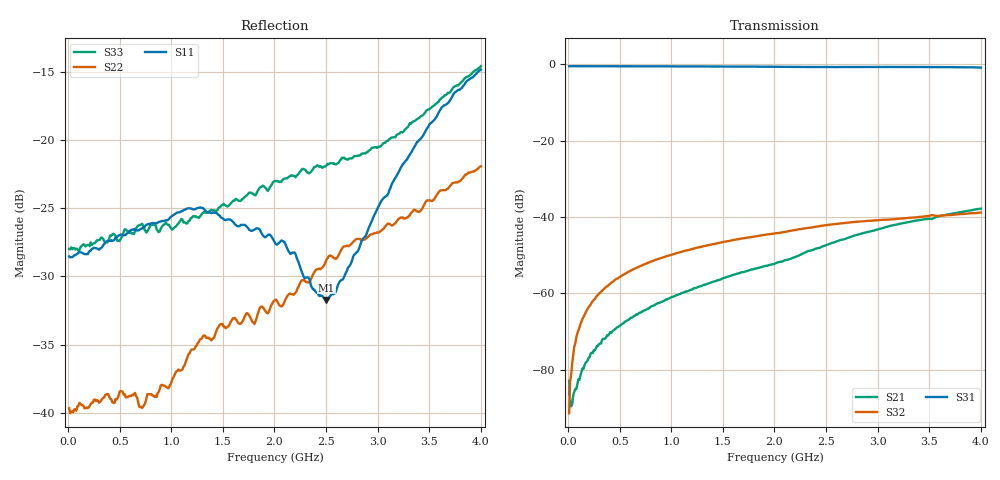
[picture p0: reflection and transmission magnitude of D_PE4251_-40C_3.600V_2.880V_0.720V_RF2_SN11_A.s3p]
! Device ID: PE4251_SoldCshunt_081809
! Dir: c:\Test Bench Repositories\Bench_Software_CVI_Version_8\trunk\PSC 4Port_VNA Bench\datalog\4250\TEST\PE4251_SoldCshunt_081809\-40C\3p600000\RF2
! Serial: 11
! Insertion: A
! Temp: -40C
! VDD: 3.600
! Control_Hi: 80.000
! Control_Lo: 20.000
! Logic State: RF2
! Port 1: RFC
! Port 2: RF1
! Port 3: RF2
! V1 = 0.72
! V2 = 0.72
! V3 = 0.72
! IDD: 4.648080e-05
! FILE NAME
! DATE 08/18/09  20:09
! CORRECTED  DATA
#  Hz  S  RI  R  50.00
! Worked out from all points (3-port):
!   401 points, 10 MHz to 4 GHz, reference 50 ohm
!   strongest paths, dB at 10 MHz, 1.008 GHz, 2.005 GHz, 3.002 GHz, 4 GHz:
!     S31: -0.5, -0.5, -0.6, -0.7, -0.8
!     S32: -91.5, -49.9, -44.3, -40.9, -38.8
!     S21: -82.9, -61.0, -52.2, -43.3, -37.8
!   lowest |S11| = -31.7 dB at 2.504 GHz (marker M1), VSWR 1.05, Z = 50.6 - j2.54 ohm
!   |S11| at or under -10 dB: start of sweep to end of sweep
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1e7  0.0375 -0.000719  4.15e-05 -6.34e-05  0.9447 -0.00293
     4.55e-05 -5.49e-05  0.0104 -0.000823  -3.47e-05 -1.77e-05
     0.9453 -0.00397  2.58e-05 6.79e-06  0.0399 0.000522
9.9775e7  0.0385 0.00196  1.14e-05 -6.84e-05  0.9445 -0.0364
          1.05e-05 -7.37e-05  0.0106 0.000318  3.18e-05 0.000321
          0.9454 -0.0359  5.07e-05 0.000322  0.0393 -5.74e-06
1.59625e8  0.0381 0.00299  -2.65e-06 -0.000117  0.9427 -0.0557
           -3.9e-06 -0.000114  0.0103 0.0013  3.71e-05 0.000525
           0.9438 -0.0562  3.87e-05 0.00052  0.0412 0.00151
4.6885e8  0.0436 0.00607  -0.000174 -0.000309  0.9296 -0.1626
          -0.000164 -0.000313  0.0107 0.00314  0.000125 0.00153
          0.9305 -0.1624  0.000133 0.00154  0.0433 -0.00308
7.18225e8  0.0473 0.00232  -0.000389 -0.000419  0.9102 -0.2441
           -0.000388 -0.000425  0.00972 0.00377  0.000278 0.0023
           0.9113 -0.2444  0.000277 0.00231  0.0491 -0.00519
1.2868e9  0.056 -0.00844  -0.00112 -0.000545  0.8375 -0.4215
          -0.00111 -0.000555  0.0167 0.00827  0.000709 0.00399
          0.8401 -0.4219  0.000696 0.004  0.0524 -0.00851
2.005e9  0.038 -0.018  -0.00233 -0.000753  0.7025 -0.6069
         -0.00232 -0.000759  0.0162 0.0202  0.00127 0.00597
         0.7041 -0.6071  0.00126 0.00597  0.065 -0.0282
2.50375e9  0.00648 -0.0251  -0.00409 -0.00126  0.5918 -0.706
           -0.0041 -0.00125  0.0183 0.0315  0.00174 0.00761
           0.5943 -0.7059  0.00175 0.00761  0.0531 -0.0609
3.38155e9  -0.0908 -0.0381  -0.00902 0.000228  0.3574 -0.8501
           -0.00899 0.000243  -0.0014 0.0548  0.00267 0.00954
           0.3587 -0.8508  0.00265 0.00954  -0.0203 -0.1177
4e9  -0.1801 -0.022  -0.0127 0.00258  0.1377 -0.8969
     -0.0126 0.00256  -0.0297 0.0745  0.00287 0.011
     0.1395 -0.8962  0.00286 0.0111  -0.1278 -0.1362
